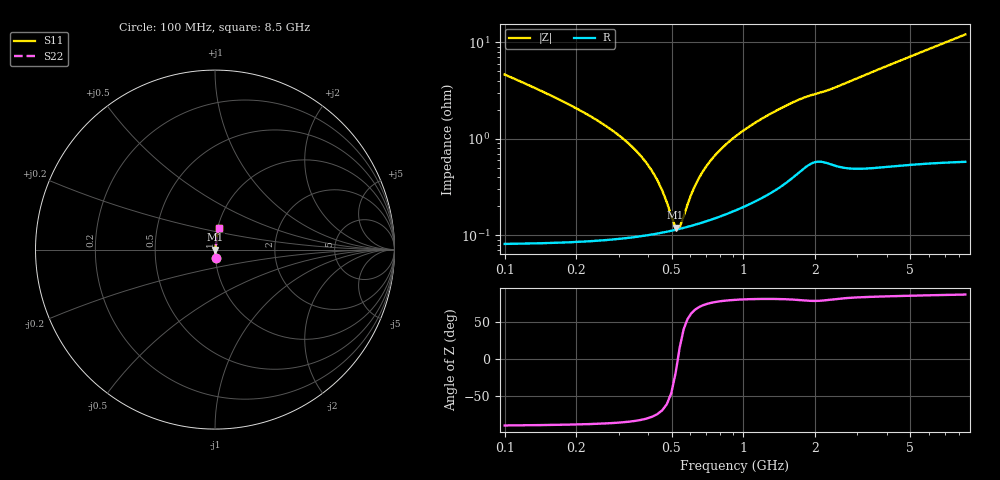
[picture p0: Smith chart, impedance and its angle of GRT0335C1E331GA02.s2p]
!Murata Part Number: GRT0335C1E331GA02
!These Parameters are Measured in Series Mode Connection
!Data Generated on Jun 19, 2026
!  o--ll--o
!Port1  Port2
!  o------o
!Operation Temp=25[degC], DC Bias Voltage=0[V]
!Freq. Start=100[MHz] Stop=9[GHz] 401[Steps]
# Hz S RI R 50
!Freq.(Hz) S11(Real) S11(Imag) S21(Real) S21(Imag) S12(Real) S12(Imag) S22(Real) S22(Imag)
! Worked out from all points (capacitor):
!   401 points, 100 MHz to 8.5 GHz, reference 50 ohm
!   read as one part in series: C = 330 pF near 142 MHz
!   lowest |Z| = 120 mohm at 520 MHz (marker M1)
!   series resonance near 531.1 MHz, so ESL is about 270 pH
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1e8  0.00297 -0.0463  0.997 0.0463  0.997 0.0463  0.00297 -0.0463
1.42e8  0.00182 -0.0314  0.9982 0.0314  0.9982 0.0314  0.00182 -0.0314
1.84e8  0.00137 -0.023  0.9986 0.023  0.9986 0.023  0.00137 -0.023
3.73e8  0.00102 -0.00652  0.999 0.00652  0.999 0.00652  0.00102 -0.00652
4.36e8  0.00105 -0.00358  0.9989 0.00358  0.9989 0.00358  0.00105 -0.00358
4.99e8  0.00112 -0.00112  0.9989 0.00112  0.9989 0.00112  0.00112 -0.00112
5.2e8  0.00114 -0.000378  0.9989 0.000378  0.9989 0.000378  0.00114 -0.000378
5.41e8  0.00117 0.000335  0.9988 -0.000335  0.9988 -0.000335  0.00117 0.000335
5.62e8  0.0012 0.00102  0.9988 -0.00102  0.9988 -0.00102  0.0012 0.00102
6.25e8  0.00129 0.00294  0.9987 -0.00294  0.9987 -0.00294  0.00129 0.00294
6.88e8  0.0014 0.0047  0.9986 -0.0047  0.9986 -0.0047  0.0014 0.0047
7.51e8  0.00152 0.00633  0.9985 -0.00633  0.9985 -0.00633  0.00152 0.00633
8.35e8  0.0017 0.00836  0.9983 -0.00836  0.9983 -0.00836  0.0017 0.00836
9.61e8  0.00201 0.0112  0.998 -0.0112  0.998 -0.0112  0.00201 0.0112
1.108e9  0.00241 0.0142  0.9976 -0.0142  0.9976 -0.0142  0.00241 0.0142
1.507e9  0.00395 0.0217  0.9961 -0.0217  0.9961 -0.0217  0.00395 0.0217
1.864e9  0.006 0.0269  0.994 -0.0269  0.994 -0.0269  0.006 0.0269
2.914e9  0.00654 0.0406  0.9935 -0.0406  0.9935 -0.0406  0.00654 0.0406
4.3e9  0.00887 0.0604  0.9911 -0.0604  0.9911 -0.0604  0.00887 0.0604
5.707e9  0.0119 0.0799  0.9881 -0.0799  0.9881 -0.0799  0.0119 0.0799
7.114e9  0.0156 0.0991  0.9844 -0.0991  0.9844 -0.0991  0.0156 0.0991
8.5e9  0.0199 0.1178  0.9801 -0.1178  0.9801 -0.1178  0.0199 0.1178
